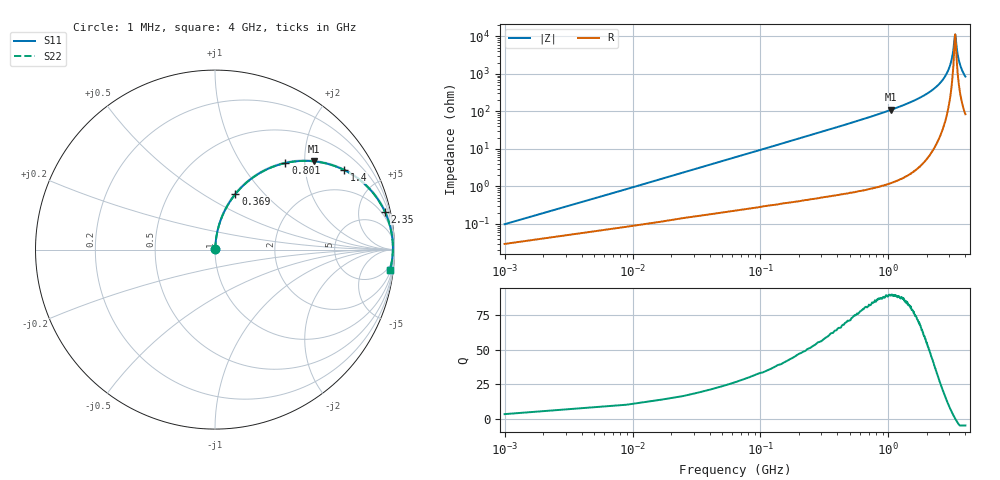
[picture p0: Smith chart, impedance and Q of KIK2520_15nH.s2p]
!version-2
!date-01.2022
!Series
# MHz S RI R 50
!Freq ReS11 ImS11 ReS21 ImS21 ReS12 ImS12 ReS22 ImS22
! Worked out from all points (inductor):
!   501 points, 1 MHz to 4 GHz, reference 50 ohm
!   read as one part in series: L = 15 nH near 17 MHz
!   highest Q = 89.5 at 1.055 GHz (marker M1), where L = 16.7 nH
!   self-resonance near 3.32 GHz
!   S11 on the Smith chart (normalised r, x): 1 MHz: 1.00, +0.00; 369 MHz: 1.01, +0.70; 801 MHz: 1.02, +1.60; 1.4 GHz: 1.04, +3.21; 2.35 GHz: 1.25, +8.86; 4 GHz: 3, -17
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1  0.000291 0.000942  0.9997 -0.000942  0.9997 -0.000942  0.000291 0.000942
25  0.00198 0.0235  0.998 -0.0235  0.998 -0.0235  0.00198 0.0235
33  0.00261 0.031  0.9974 -0.031  0.9974 -0.031  0.00261 0.031
81  0.00833 0.0756  0.9917 -0.0756  0.9917 -0.0756  0.00833 0.0756
193  0.0358 0.1753  0.9642 -0.1753  0.9642 -0.1753  0.0358 0.1753
369  0.1142 0.3101  0.8858 -0.3101  0.8858 -0.3101  0.1142 0.3101
673  0.3065 0.4549  0.6935 -0.4549  0.6935 -0.4549  0.3065 0.4549
801  0.3923 0.4824  0.6077 -0.4824  0.6077 -0.4824  0.3923 0.4824
1055  0.5505 0.4919  0.4495 -0.4919  0.4495 -0.4919  0.5505 0.4919
1335  0.691 0.4563  0.309 -0.4563  0.309 -0.4563  0.691 0.4563
1400  0.718 0.4441  0.282 -0.4441  0.282 -0.4441  0.718 0.4441
2010  0.8943 0.2983  0.1057 -0.2983  0.1057 -0.2983  0.8943 0.2983
2350  0.9461 0.212  0.0539 -0.212  0.0539 -0.212  0.9461 0.212
2670  0.974 0.1363  0.026 -0.1363  0.026 -0.1363  0.974 0.1363
3100  0.9899 0.0451  0.0101 -0.0451  0.0101 -0.0451  0.9899 0.0451
3220  0.9911 0.0213  0.00894 -0.0213  0.00894 -0.0213  0.9911 0.0213
3310  0.9912 0.00292  0.00881 -0.00292  0.00881 -0.00292  0.9912 0.00292
3340  0.9911 -0.0016  0.00889 0.0016  0.00889 0.0016  0.9911 -0.0016
3430  0.9904 -0.0193  0.00962 0.0193  0.00962 0.0193  0.9904 -0.0193
3550  0.9886 -0.0408  0.0114 0.0408  0.0114 0.0408  0.9886 -0.0408
3750  0.9838 -0.0746  0.0162 0.0746  0.0162 0.0746  0.9838 -0.0746
4000  0.9752 -0.1135  0.0248 0.1135  0.0248 0.1135  0.9752 -0.1135
